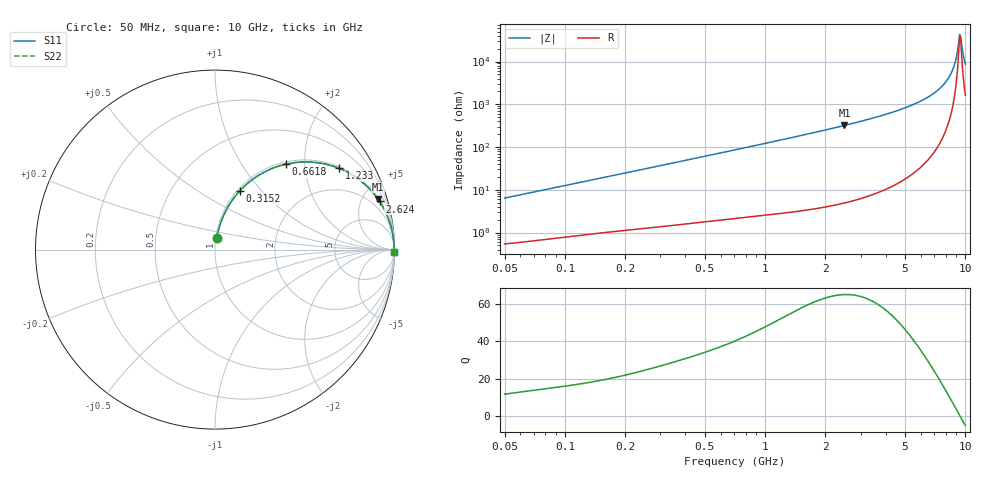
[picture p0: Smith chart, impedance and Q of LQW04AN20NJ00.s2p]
!Murata Part Number: LQW04AN20NJ00
!These Parameters are Measured in Series Mode Connection
!  o--[Z]--o
!Port1  Port2
!  o-------o
!Freq. Start=50[MHz] Stop=10[GHz], 401[Steps]
# Hz S RI R 50
!Freq.(Hz)	S 11(Real)	S 11(Imag)	S 21(Real)	S 21(Imag)	S 12(Real)	S 12(Imag)	S 22(Real)	S 22(Imag)
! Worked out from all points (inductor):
!   401 points, 50 MHz to 10 GHz, reference 50 ohm
!   read as one part in series: L = 20.2 nH near 51.34 MHz
!   highest Q = 65.1 at 2.489 GHz (marker M1), where L = 20.5 nH
!   self-resonance near 9.359 GHz
!   S11 on the Smith chart (normalised r, x): 50 MHz: 1.01, +0.13; 315.2 MHz: 1.03, +0.77; 661.8 MHz: 1.04, +1.61; 1.233 GHz: 1.06, +3.02; 2.624 GHz: 1.10, +6.80; 10 GHz: open
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5e7  0.0094 0.0629  0.9906 -0.0629  0.9906 -0.0629  0.0094 0.0629
1.214486e8  0.0306 0.1459  0.9694 -0.1459  0.9694 -0.1459  0.0306 0.1459
2.949953e8  0.1247 0.3122  0.8753 -0.3122  0.8753 -0.3122  0.1247 0.3122
3.15194e8  0.1386 0.3278  0.8614 -0.3278  0.8614 -0.3278  0.1386 0.3278
6.617929e8  0.3956 0.4763  0.6044 -0.4763  0.6044 -0.4763  0.3956 0.4763
7.071068e8  0.4267 0.4823  0.5733 -0.4823  0.5733 -0.4823  0.4267 0.4823
1.233369e9  0.6912 0.4526  0.3088 -0.4526  0.3088 -0.4526  0.6912 0.4526
1.717543e9  0.8154 0.3798  0.1846 -0.3798  0.1846 -0.3798  0.8154 0.3798
2.488741e9  0.9075 0.2822  0.0925 -0.2822  0.0925 -0.2822  0.9075 0.2822
2.624158e9  0.917 0.2683  0.083 -0.2683  0.083 -0.2683  0.917 0.2683
4.171863e9  0.9718 0.1567  0.0282 -0.1567  0.0282 -0.1567  0.9718 0.1567
6.045081e9  0.991 0.0811  0.00901 -0.0811  0.00901 -0.0811  0.991 0.0811
7.571744e9  0.9962 0.0393  0.00376 -0.0393  0.00376 -0.0393  0.9962 0.0393
8.090191e9  0.9971 0.0273  0.00292 -0.0273  0.00292 -0.0273  0.9971 0.0273
8.530394e9  0.9975 0.0177  0.00247 -0.0177  0.00247 -0.0177  0.9975 0.0177
8.876195e9  0.9977 0.0105  0.00226 -0.0105  0.00226 -0.0105  0.9977 0.0105
9.236013e9  0.9978 0.0033  0.00216 -0.0033  0.00216 -0.0033  0.9978 0.0033
9.359165e9  0.9979 0.000891  0.00215 -0.000891  0.00215 -0.000891  0.9979 0.000891
9.48396e9  0.9979 -0.00153  0.00215 0.00153  0.00215 0.00153  0.9979 -0.00153
9.610418e9  0.9978 -0.00395  0.00216 0.00395  0.00216 0.00395  0.9978 -0.00395
9.868415e9  0.9978 -0.00882  0.00223 0.00882  0.00223 0.00882  0.9978 -0.00882
1e10  0.9977 -0.0113  0.00228 0.0113  0.00228 0.0113  0.9977 -0.0113
